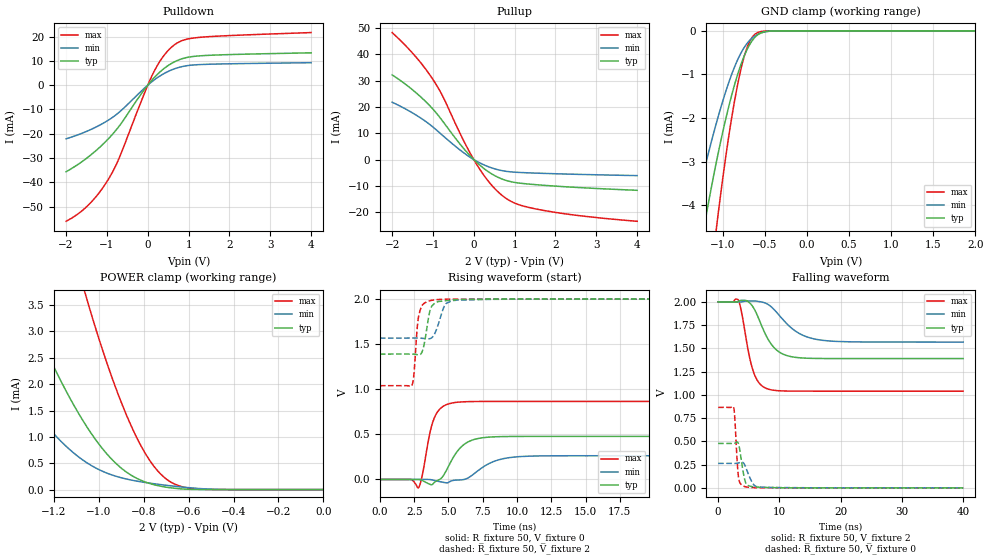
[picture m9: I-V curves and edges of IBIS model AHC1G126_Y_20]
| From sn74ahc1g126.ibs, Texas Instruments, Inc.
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[Model]   AHC1G126_Y_20
Model_type  3-state
Enable   Active-High
Vref =   0
Rref =   1000
Cref =   50p
Vmeas =   1.0
| variable   typ   min   max
C_comp   2.95pF   2.48pF   3.17pF
| C_pullup   4.07pF   2.71pF   4.98pF
| C_pulldown   5.18pF   3.21pF   8.35pF
| C_tri-state   2.95pF   2.48pF   3.17pF
[Temperature Range]   40   100   -40
| Ambient temperature   25   85   -40
[Voltage range]   2   2   2
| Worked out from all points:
|   slope of the pulldown table from 0 to 0.3 V, typ, clamps not added: 55 ohm
|   slope of the pullup table from 0 to 0.3 V, typ, clamps not added: 74.8 ohm
|   GND clamp passes 1 mA (typ) near -0.82 V on its own axis
|   POWER clamp passes 1 mA (typ) near -1.02 V on its own axis
|   rising waveform, R_fixture 50, V_fixture 0: 20-80 % time 1.26ns typ, 1.74ns min, 751ps max; typ from 0 V to 0.478 V
|   falling waveform, R_fixture 50, V_fixture 2: 20-80 % time 2.84ns typ, 4.23ns min, 1.8ns max; typ from 2 V to 1.39 V
|   rising waveform, R_fixture 50, V_fixture 2: 20-80 % time 416ps typ, 567ps min, 308ps max; typ from 1.39 V to 2 V
|   falling waveform, R_fixture 50, V_fixture 0: 20-80 % time 723ps typ, 1.05ns min, 460ps max; typ from 0.478 V to 0 V
[GND Clamp]
| AHC1G126_Y_20
|   Voltage   I(typ)   I(min)   I(max)
-2V       -15.54mA   -10.83mA   -25.02mA
-1.38V    -6.369mA   -4.535mA   -10.17mA
-1.36V    -6.122mA   -4.36mA    -9.76mA
-1.22V    -4.495mA   -3.196mA   -7.031mA
-1.2V     -4.277mA   -3.039mA   -6.665mA
-1.07V    -2.961mA   -2.08mA    -4.453mA
-935mV    -1.79mA    -1.224mA   -2.506mA
-810mV    -923.9uA   -611.5uA   -1.112mA
-705mV    -406.5uA   -274.6uA   -353.7uA
-600mV    -115.8uA   -96.74uA   -55.88uA
-385mV    -2.171uA   -2.811uA   -254.8nA
2V        142.1pA    583.4pA    2.536pA
[POWER Clamp]
| AHC1G126_Y_20
|   Voltage   I(typ)   I(min)   I(max)
-2V       12.67mA    7.242mA    24.62mA
-1.6V     6.742mA    3.612mA    14.28mA
-1.335V   3.625mA    1.777mA    8.507mA
-1.2V     2.33mA     1.058mA    5.982mA
-1.065V   1.272mA    543.8uA    3.791mA
-1.05V    1.172mA    501.4uA    3.571mA
-965mV    683.1uA    315.2uA    2.418mA
-865mV    298.5uA    190uA      1.299mA
-785mV    132.1uA    129.9uA    631.8uA
-710mV    53.03uA    87.3uA     237.8uA
-565mV    2.679uA    24.45uA    12.95uA
-20.5fV   142.1pA    583.4pA    2.536pA
[Pulldown]
| AHC1G126_Y_20
|   Voltage   I(typ)   I(min)   I(max)
-2V       -35.64mA   -22.08mA   -56.02mA
-1.45V    -29.46mA   -18.67mA   -49.26mA
-1.2V     -25.92mA   -16.66mA   -44.49mA
-970mV    -22.15mA   -14.45mA   -38.88mA
-695mV    -16.75mA   -11.06mA   -29.79mA
-125mV    -2.781mA   -1.912mA   -5.145mA
115mV     2.311mA    1.603mA    4.288mA
370mV     6.465mA    4.507mA    11.62mA
635mV     9.44mA     6.61mA     16.38mA
885mV     11.09mA    7.792mA    18.59mA
1.26V     12.05mA    8.457mA    19.66mA
4V        13.31mA    9.244mA    21.64mA
[Pullup]
| AHC1G126_Y_20
|   Voltage   I(typ)   I(min)   I(max)
-2V       32.22mA    21.8mA     48.31mA
-1.465V   26.09mA    17.41mA    39.89mA
-1.04V    19.87mA    12.88mA    31.39mA
-775mV    14.88mA    9.343mA    24.54mA
-285mV    4.911mA    3.026mA    8.317mA
45mV      -679.6uA   -407uA     -1.181mA
385mV     -4.919mA   -2.876mA   -8.785mA
720mV     -7.563mA   -4.289mA   -13.96mA
1.07V     -8.852mA   -4.86mA    -16.98mA
1.64V     -9.7mA     -5.219mA   -19.15mA
2.64V     -10.7mA    -5.658mA   -21.43mA
4V        -11.69mA   -6.099mA   -23.48mA
[Ramp]
| AHC1G126_Y_20
| variable   typ   min   max
dV/dt_r   0.32/1.34E-09   0.18/1.88E-09   0.57/7.87E-10
dV/dt_f   0.38/2.89E-09   0.27/4.29E-09   0.59/1.84E-09
R_load = 50
[Rising Waveform]
| AHC1G126_Y_20
R_fixture =   50
C_fixture =   0
L_fixture =   0
V_fixture =   0
V_fixture_min = 0
V_fixture_max = 0
|   Time   V(typ)   V(min)   V(max)
0s        103.5pV    209.5pV    42.13pV
2.29ns    113.1uV    -37.46uV   -258.3uV
2.825ns   832.1uV    432.6uV    -89.91mV
3.985ns   -31.08mV   -10.88mV   687.2mV
4.59ns    33.39mV    -30.26mV   808.3mV
5.465ns   272.1mV    -7.721mV   853mV
6.945ns   446.5mV    72.34mV    864.7mV
8.445ns   473.6mV    207.4mV    865.7mV
10.45ns   477.5mV    255.7mV    865.7mV
40ns      477.7mV    263.4mV    865.8mV
[Falling Waveform]
| AHC1G126_Y_20
R_fixture =   50
C_fixture =   0
L_fixture =   0
V_fixture =   2
V_fixture_min = 2
V_fixture_max = 2
|   Time   V(typ)   V(min)   V(max)
0s        2V         2V         2V
3.305ns   2.006V     1.999V     2.018V
4.59ns    2.015V     2.009V     1.597V
5.695ns   1.945V     2.01V      1.262V
6.665ns   1.813V     2.004V     1.13V
8.01ns    1.615V     1.978V     1.066V
10.7ns    1.435V     1.801V     1.042V
13.11ns   1.4V       1.666V     1.04V
15.95ns   1.392V     1.598V     1.04V
40ns      1.391V     1.568V     1.04V
[Rising Waveform]
| AHC1G126_Y_20
R_fixture =   50
C_fixture =   0
L_fixture =   0
V_fixture =   2
V_fixture_min = 2
V_fixture_max = 2
|   Time   V(typ)   V(min)   V(max)
0s        1.391V     1.568V     1.04V
2.315ns   1.391V     1.569V     1.037V
2.465ns   1.39V      1.569V     1.142V
2.75ns    1.383V     1.569V     1.722V
2.91ns    1.383V     1.568V     1.861V
3.655ns   1.873V     1.562V     1.982V
3.905ns   1.941V     1.592V     1.99V
4.755ns   1.982V     1.938V     1.999V
5.635ns   1.994V     1.988V     2V
40ns      2V         2V         2V
[Falling Waveform]
| AHC1G126_Y_20
R_fixture =   50
C_fixture =   0
L_fixture =   0
V_fixture =   0
V_fixture_min = 0
V_fixture_max = 0
|   Time   V(typ)   V(min)   V(max)
0s        477.7mV    263.4mV    865.8mV
2.53ns    477.5mV    262.8mV    866.6mV
2.7ns     480.8mV    262.7mV    770.5mV
3.105ns   493.1mV    264.7mV    289.1mV
3.33ns    471mV      268mV      112.8mV
4.245ns   116.9mV    257.8mV    15.74mV
4.645ns   36.07mV    197.2mV    9.558mV
5.675ns   12.05mV    46.05mV    3.011mV
6.745ns   6.872mV    9.513mV    960.7uV
40ns      136.7pV    90.4nV     41.78pV
